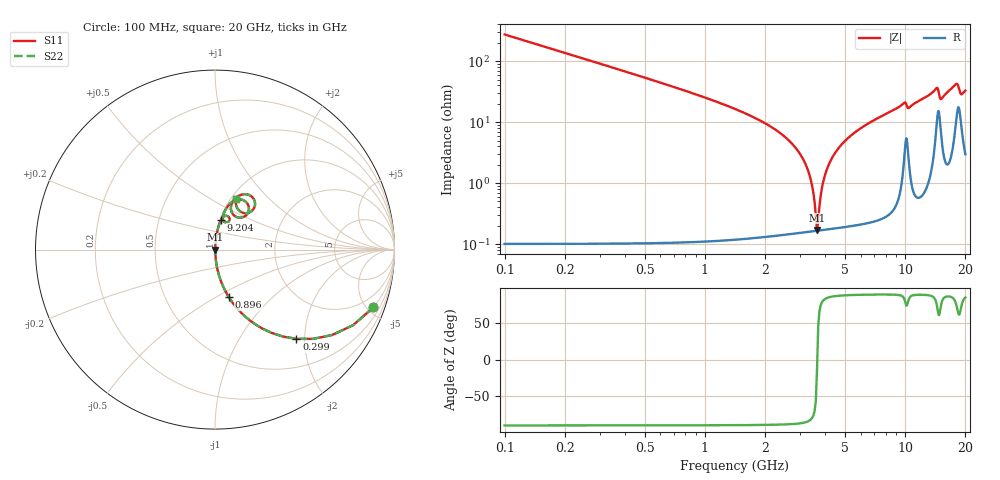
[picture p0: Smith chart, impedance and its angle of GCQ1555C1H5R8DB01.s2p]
!Murata Part Number: GCQ1555C1H5R8DB01
!These Parameters are Measured in Series Mode Connection
!Data Generated on Mar 13, 2026
!  o--ll--o
!Port1  Port2
!  o------o
!Operation Temp=25[degC], DC Bias Voltage=0[V]
!Freq. Start=100[MHz] Stop=20[GHz] 401[Steps]
# Hz S RI R 50
!Freq.(Hz) S11(Real) S11(Imag) S21(Real) S21(Imag) S12(Real) S12(Imag) S22(Real) S22(Imag)
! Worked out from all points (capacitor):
!   401 points, 100 MHz to 20 GHz, reference 50 ohm
!   read as one part in series: C = 5.8 pF near 199.5 MHz
!   lowest |Z| = 170 mohm at 3.632 GHz (marker M1)
!   series resonance near 3.642 GHz, so ESL is about 330 pH
!   S11 on the Smith chart (normalised r, x): 100 MHz: 1.00, -5.48; 299 MHz: 1.00, -1.82; 896 MHz: 1.00, -0.58; 9.204 GHz: 1.01, +0.35; 20 GHz: 1.06, +0.66
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1e8  0.8825 -0.3218  0.1175 0.3218  0.1175 0.3218  0.8825 -0.3218
2.99e8  0.4539 -0.4973  0.5461 0.4973  0.5461 0.4973  0.4539 -0.4973
5.4775e8  0.1939 -0.3943  0.8061 0.3943  0.8061 0.3943  0.1939 -0.3943
8.96e8  0.0773 -0.2651  0.9227 0.2651  0.9227 0.2651  0.0773 -0.2651
2.7865e9  0.00314 -0.0406  0.9969 0.0406  0.9969 0.0406  0.00314 -0.0406
3.1845e9  0.00197 -0.0202  0.998 0.0202  0.998 0.0202  0.00197 -0.0202
3.43325e9  0.00169 -0.00886  0.9983 0.00886  0.9983 0.00886  0.00169 -0.00886
3.63225e9  0.00165 -0.000382  0.9983 0.000382  0.9983 0.000382  0.00165 -0.000382
3.9805e9  0.0019 0.0134  0.9981 -0.0134  0.9981 -0.0134  0.0019 0.0134
4.478e9  0.00279 0.0314  0.9972 -0.0314  0.9972 -0.0314  0.00279 0.0314
5.3735e9  0.00561 0.0602  0.9944 -0.0602  0.9944 -0.0602  0.00561 0.0602
6.7665e9  0.0124 0.0998  0.9876 -0.0998  0.9876 -0.0998  0.0124 0.0998
9.20425e9  0.0339 0.1666  0.9661 -0.1666  0.9661 -0.1666  0.0339 0.1666
1.005e10  0.0789 0.1788  0.9211 -0.1788  0.9211 -0.1788  0.0789 0.1788
1.039825e10  0.0507 0.1558  0.9493 -0.1558  0.9493 -0.1558  0.0507 0.1558
1.338325e10  0.0875 0.2598  0.9125 -0.2598  0.9125 -0.2598  0.0875 0.2598
1.437825e10  0.1705 0.2674  0.8295 -0.2674  0.8295 -0.2674  0.1705 0.2674
1.507475e10  0.1067 0.1897  0.8933 -0.1897  0.8933 -0.1897  0.1067 0.1897
1.67165e10  0.1172 0.289  0.8828 -0.289  0.8828 -0.289  0.1172 0.289
1.83085e10  0.2232 0.2535  0.7768 -0.2535  0.7768 -0.2535  0.2232 0.2535
1.895525e10  0.147 0.2088  0.853 -0.2088  0.853 -0.2088  0.147 0.2088
2e10  0.1185 0.281  0.8815 -0.281  0.8815 -0.281  0.1185 0.281
